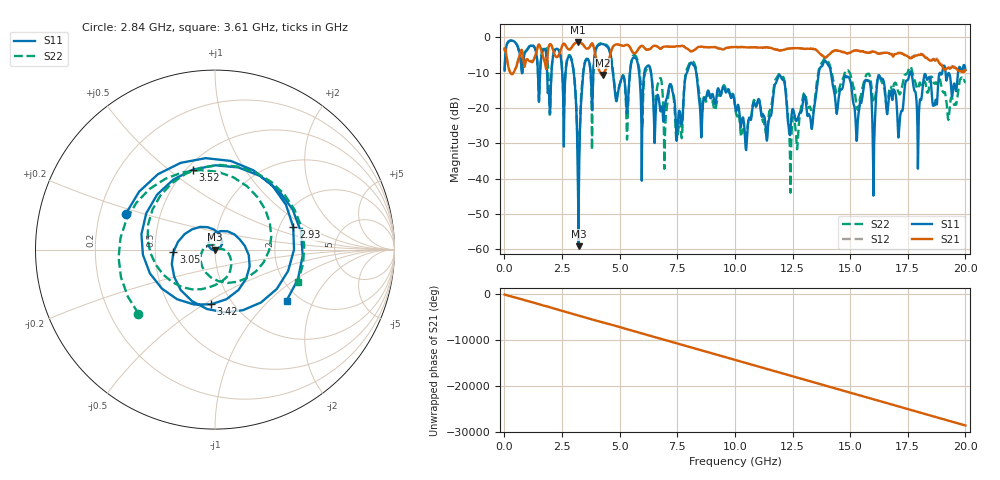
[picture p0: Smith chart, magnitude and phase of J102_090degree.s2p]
!Keysight Technologies,N5222A,MY51421036,A.10.65.16
!Date: Friday, March 31, 2023 14:54:17
!Correction: S11(Full 2 Port(1,2))
!S21(Full 2 Port(1,2))
!S12(Full 2 Port(1,2))
!S22(Full 2 Port(1,2))
!S2P File: Measurements: S11, S21, S12, S22:
# Hz S  dB  R 50
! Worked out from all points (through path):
!   2000 points, 10 MHz to 20 GHz, reference 50 ohm
!   highest |S21| = -1.43 dB at 3.2 GHz (marker M1); lowest = -10.6 dB at 4.26 GHz (marker M2)
!   group delay of S21, straight-line fit = 3.98 ns
!   lowest |S11| = -59.1 dB at 3.22 GHz (marker M3), VSWR 1.00, Z = 49.9 - j0.00179 ohm
!   |S11| at or under -10 dB: 6.363 GHz to 7.92 GHz (1.558 GHz wide, 21.8 % of centre); 8.322 GHz to 13.64 GHz (5.318 GHz wide, 48.4 % of centre); 14.17 GHz to 17.59 GHz (3.423 GHz wide, 21.6 % of centre)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
!   |S22| runs from -44.0 to -0.9 dB; largest |S21 - S12| = 0.022
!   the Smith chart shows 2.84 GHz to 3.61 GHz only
!   S11 on the Smith chart (normalised r, x): 2.84 GHz: 0.31, +0.18; 2.93 GHz: 2.37, +0.76; 3.05 GHz: 0.62, -0.02; 3.42 GHz: 0.80, -0.54; 3.52 GHz: 0.54, +0.61; 3.61 GHz: 1.72, -1.29
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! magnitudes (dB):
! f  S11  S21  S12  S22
! 10 MHz  -9.4  -3.2  -3.1  -9.4
! 2.84 GHz  -5.4  -3.5  -3.4  -5.1
! 2.93 GHz  -6.9  -2.8  -2.7  -6.6
! 3.05 GHz  -12.7  -1.7  -1.7  -12.5
! 3.2 GHz  -45.7  -1.4  -1.4  -33.8
! 3.22 GHz  -59.1  -1.5  -1.4  -34.3
! 3.35 GHz  -16.5  -1.8  -1.8  -14.8
! 3.42 GHz  -10.3  -2.1  -2.1  -9.9
! 3.52 GHz  -6.7  -3.0  -3.0  -6.5
! 3.61 GHz  -6.2  -3.2  -3.2  -6.1
! 4.26 GHz  -1.9  -10.6  -10.6  -1.6
! 5.31 GHz  -21.1  -2.1  -2.1  -27.1
! 5.62 GHz  -5.7  -4.5  -4.5  -5.1
! 6.68 GHz  -16.7  -2.8  -2.8  -12.7
! 7.52 GHz  -24.8  -2.5  -2.5  -27.7
! 8.11 GHz  -7.2  -4.0  -4.0  -6.7
! 8.53 GHz  -26.4  -2.7  -2.6  -20.4
! 10.01 GHz  -19.6  -2.7  -2.7  -19.5
! 13.34 GHz  -25.9  -3.3  -3.2  -21.6
! 13.91 GHz  -6.7  -5.7  -5.6  -5.9
! 16.67 GHz  -17.8  -4.5  -4.4  -16.3
! 20 GHz  -9.2  -9.3  -9.0  -12.7
